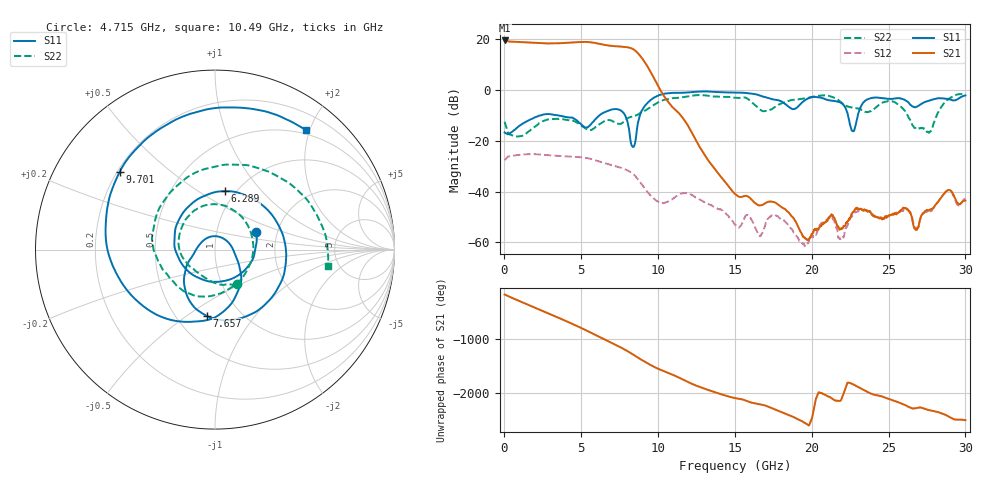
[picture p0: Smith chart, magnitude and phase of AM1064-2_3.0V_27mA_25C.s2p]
!Agilent Technologies,E8364B,MY43040894,A.07.50.67
!Agilent E8364B: A.07.50.67
!Date: Tuesday, March 05, 2019 05:08:22
!Correction: S11(Full 2 Port(1,2))
!S21(Full 2 Port(1,2))
!S12(Full 2 Port(1,2))
!S22(Full 2 Port(1,2))
!S2P File: Measurements: S11, S21, S12, S22:
# Hz S  dB  R 50
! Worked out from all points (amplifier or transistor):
!   1601 points, 10 MHz to 30 GHz, reference 50 ohm
!   highest |S21| = 19.3 dB at 10 MHz (marker M1)
!   |S21| within 3 dB of that: start of sweep to 8.225 GHz
!   unconditionally stable (mu >= 1): start of sweep to end of sweep
!   at 4.996 GHz: K = 1.38, MAG = 18.9 dB, |S12| = -26.6 dB
!   at 15.01 GHz: K = 3026.70, MAG = -31.8 dB, |S12| = -52.9 dB
!   at 30 GHz: K = 1455.80, MAG = -34.9 dB, |S12| = -42.9 dB
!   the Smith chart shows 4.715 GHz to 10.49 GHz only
!   S11 on the Smith chart (normalised r, x): 4.715 GHz: 1.55, +0.32; 6.289 GHz: 0.90, +0.65; 7.657 GHz: 0.70, -0.60; 9.701 GHz: 0.21, +0.34; 10.49 GHz: 0.44, +1.94
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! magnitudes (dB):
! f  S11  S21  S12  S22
! 10 MHz  -16.8  19.3  -27.7  -12.7
! 4.715 GHz  -12.1  18.6  -26.5  -13.0
! 5.015 GHz  -13.8  18.7  -26.6  -14.2
! 6.289 GHz  -9.6  17.8  -28.4  -13.2
! 7.657 GHz  -8.6  16.8  -30.8  -13.1
! 8.37 GHz  -22.5  15.9  -33.1  -10.7
! 9.701 GHz  -3.3  4.8  -42.7  -6.1
! 10.02 GHz  -2.3  1.2  -44.0  -5.0
! 10.49 GHz  -1.6  -3.5  -44.3  -3.9
! 12.01 GHz  -1.1  -14.8  -40.8  -2.6
! 15.01 GHz  -1.2  -40.9  -52.9  -3.2
! 16.65 GHz  -2.4  -45.4  -57.3  -7.9
! 17.63 GHz  -4.0  -44.3  -49.2  -6.8
! 20.01 GHz  -3.0  -56.6  -57.7  -2.9
! 21.21 GHz  -4.3  -49.6  -49.8  -2.6
! 21.96 GHz  -5.4  -54.4  -58.3  -5.2
! 22.69 GHz  -16.4  -47.9  -49.2  -7.2
! 23.46 GHz  -4.4  -47.3  -47.2  -8.6
! 25.01 GHz  -3.6  -49.4  -49.6  -4.6
! 26.81 GHz  -6.7  -55.0  -54.3  -15.5
! 27.62 GHz  -4.4  -47.5  -48.1  -16.9
! 30 GHz  -2.3  -43.5  -42.9  -1.8
